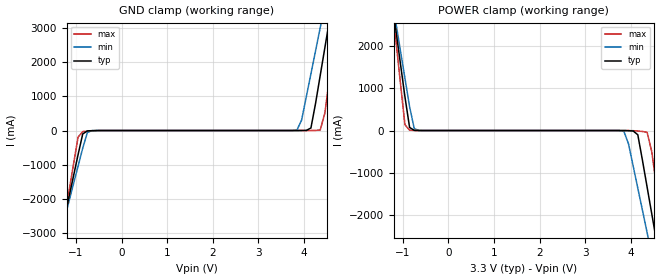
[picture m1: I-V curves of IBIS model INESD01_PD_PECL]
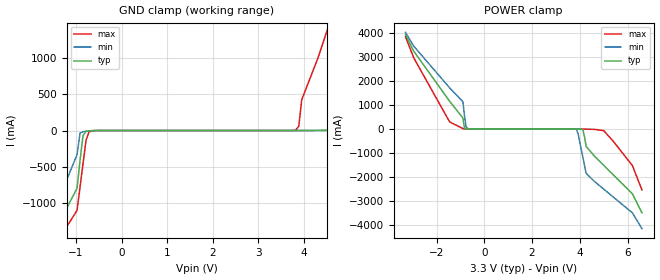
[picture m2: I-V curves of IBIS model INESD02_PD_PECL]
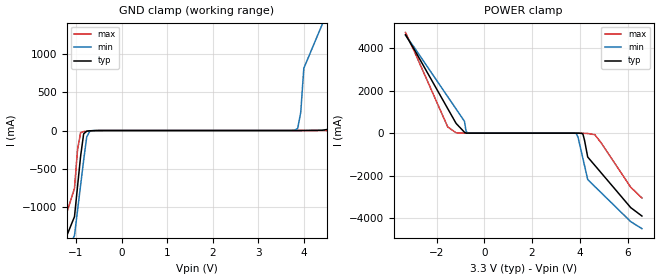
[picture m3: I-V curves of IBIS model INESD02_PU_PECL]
|   This file is an IBIS representation of the   |
|   Integrated Device Technology, Inc.   |
|   ICS8735-31   |
|   1:5 DIFFERENTIAL-TO-3.3V LVPECL ZERO DELAY CLOCK GENERATOR   |
[IBIS Ver]   4.1
[File name]   8735_31_3v3.ibs
[File Rev]   1.1
[Date]   19 Mar 2009 | Last modified
|   Dec 30 2002 | Generated
[Source]   Originated at Integrated Devices Technology, Inc.
[Disclaimer]
IDT hereby grants the user of this IBIS model a non-exclusive,
nontransferable license to use this IBIS model under the following terms.
Before using this IBIS model, the user should read this license.
If the user does not accept these terms,  the IBIS model should be
returned to IDT within 30 days.
   The user is granted this license only to use the IBIS model and
is not granted rights to sell, load, rent, lease or license the IBIS
model in whole or in part, or in modified form to anyone other than
user. User may modify the IBIS model to suit its specific
applications but rights to derivative works and such modifications
shall belong to IDT.
   This IBIS model is provided on an "AS IS" basis and IDT makes
absolutely no warranty with respect to the information contained
herein. IDT DISCLAIMS AND CUSTOMER WAIVES ALL WARRANTIES, EXPRESS
OR IMPLIED, INCLUDING WARRANTIES OF MERCHANTABILITY OR FITNESS FOR
A PARTICULAR PURPOSE. The entire risk as to quality and performance
is with the Customer. ACCORDINGLY, IN NO EVENT SHALL THE COMPANY BE
LIABLE FOR ANY DAMAGES, WHETHER IN CONTRACT OR TORT,INCLUDING ANY
LOST PROFITS OR OTHER INCIDENTAL, CONSEQUENTIAL, EXEMPLARY, OR
PUNITIVE DAMAGES ARISING OUT OF THE USE OR APPLICATION OF THE IBIS
model provided in this package. Further, IDT reserves the right to
make changes without notice to any product herein to improve
reliability, function, or design. IDT does not convey any license
under patent rights or any other intellectual property rights,
including those of third parties.
   IDT is not obligated to provide maintenance or support
for the licensed IBIS model.
[Copyright]   Copyright 2008 by Integrated Device Technology, Inc.
[Component]   ICS8735Y-31
[Manufacturer] Integrated Devices Technology, Inc.
[Package]
|LQFP32
|lead + wire   typ   min   max
R_pkg   220.4m   212.5m   238m
L_pkg   1.841n   1.708n   1.974n
C_pkg   0.316p   0.2907p   0.33p
[Pin] signal_name  model_name   R_pin   L_pin   C_pin
1   SEL0   INESD01_PD_PECL   238m   1.974n   0.330p
2   SEL1   INESD01_PD_PECL   225m   1.841n   0.311p
3   CLK0   INESD02_PD_PECL   218m   1.7745n   0.301p
4   nCLK0   INESD02_PU_PECL   213m   1.708n   0.291p
5   CLK1   INESD02_PD_PECL   213m   1.708n   0.291p
6   nCLK1   INESD02_PU_PECL   218m   1.7745n   0.301p
7   CLK_SEL   INESD01_PD_PECL   225m   1.841n   0.311p
8   MR   INESD01_PD_PECL   238m   1.974n   0.330p
9   VCC   POWER   238m   1.974n   0.330p
10   FB_IN   INESD02_PU_PECL   225m   1.841n   0.311p
11   nFB_IN   INESD02_PD_PECL   218m   1.7745n   0.301p
12   SEL2   INESD01_PD_PECL   213m   1.708n   0.291p
13   VEE   GND   213m   1.708n   0.291p
14   nQ0   ONF01_HSTL01   218m   1.7745n   0.301p
15   Q0   ONF01_HSTL01   225m   1.841n   0.311p
16   VCCO   POWER   238m   1.974n   0.330p
17   VCCO   POWER   238m   1.974n   0.330p
18   nQ1   ONF01_HSTL01   225m   1.841n   0.311p
19   Q1   ONF01_HSTL01   218m   1.7745n   0.301p
20   nQ2   ONF01_HSTL01   213m   1.708n   0.291p
21   Q2   ONF01_HSTL01   213m   1.708n   0.291p
22   nQ3   ONF01_HSTL01   218m   1.7745n   0.301p
23   Q3   ONF01_HSTL01   225m   1.841n   0.311p
24   VCCO   POWER   238m   1.974n   0.330p
25   VCCO   POWER   238m   1.974n   0.330p
26   nQ4   ONF01_HSTL01   225m   1.841n   0.311p
27   Q4   ONF01_HSTL01   218m   1.7745n   0.301p
28   VEE   GND   213m   1.708n   0.291p
29   SEL3   INESD01_PD_PECL   213m   1.708n   0.291p
30   VCCA   POWER   218m   1.7745n   0.301p
31   PLL_SEL   INESD01_PU_PECL   225m   1.841n   0.311p
32   VCC   POWER   238m   1.974n   0.330p
[Diff Pin]  inv_pin  vdiff tdelay_typ tdelay_min  tdelay_max
|Input
3   4   0.15 0  0  0
5   6   0.15 0  0  0
10   11  0.15 0  0  0
|Output
15   14   NA   0  0  0
19   18   NA   0  0  0
21   20   NA   0  0  0
23   22   NA   0  0  0
27   26   NA   0  0  0
| Models and submodels in the file (5): INESD01_PD_PECL (Input), INESD02_PD_PECL (Input), INESD02_PU_PECL (Input), ONF01_HSTL01 (Output_ECL), INESD01_PU_PECL (Input)
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[Model]   INESD01_PD_PECL
Model_type  Input
Polarity   Non-Inverting
Vinl = 0.8V
Vinh = 2.0V
|   typ   min   max
C_comp   2pF   1.5pF   2.5pF
|   typ   min   max
[Voltage range]  3.3V   3.15V   3.45V
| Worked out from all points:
|   GND clamp passes 1 mA (typ) near -0.55 V on its own axis
|   POWER clamp passes 1 mA (typ) near -0.66 V on its own axis
[GND_clamp]
|Voltage   I(typ)   I(min)   I(max)
-2.586V   -10.86A    -9.487A    -13.15A
-1.361V   -3.24A     -3.145A    -3.432A
-1.259V   -2.606A    -2.617A    -2.622A
-952.6mV  -705.3mA   -1.038A    -192.4mA
-850.5mV  -99.9mA    -513.5mA   -31.23mA
-646.4mV  -3.788mA   -3.549mA   -8.297mA
3.844V    129.1uA    13.13mA    71.12uA
4.151V    73.33mA    1.652A     864.7uA
4.355V    1.607A     3.003A     15.44mA
4.559V    3.233A     4.356A     1.553A
4.763V    4.861A     5.711A     3.635A
5.375V    9.757A     9.783A     9.893A
[POWER_clamp]
|Voltage   I(typ)   I(min)   I(max)
-2.177V   10.57A     9.364A     12.62A
-1.157V   2.42A      2.586A     2.194A
-952.6mV  795.8mA    1.237A     137.8mA
-850.5mV  73.33mA    563.2mA    8.145mA
-646.4mV  535.8uA    2.004mA    431.2uA
3.844V    -826.3uA   -18.14mA   -47.07uA
4.151V    -99.9mA    -1.362A    -11.82mA
4.355V    -1.338A    -2.415A    -41.71mA
4.559V    -2.606A    -3.47A     -1.312A
4.661V    -3.24A     -3.998A    -2.123A
4.763V    -3.875A    -4.526A    -2.933A
5.579V    -8.954A    -8.756A    -9.414A
[Model]   INESD02_PD_PECL
Model_type  Input
Polarity   Non-Inverting
Vinl = 0.8V
Vinh = 2.0V
|   typ   min   max
C_comp   2pF   1.5pF   2.5pF
|   typ   min   max
[Voltage range]  3.3V   3.15V   3.45V
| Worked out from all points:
|   GND clamp passes 1 mA (typ) near -0.59 V on its own axis
|   POWER clamp passes 1 mA (typ) near -0.70 V on its own axis
[GND_clamp]
-3.3V     -3.894A    -4.294A    -3.674A
-1.6V     -1.569A    -1.322A    -1.74A
-974.8mV  -794.1mA   -331.5mA   -1.096A
-843.4mV  -68.33mA   -15.34mA   -452.9mA
-646.5mV  -1.912mA   -4.151mA   -2.665mA
3.818V    89.38uA    70.49uA    7.198mA
3.95V     342.2uA    75.94uA    423.8mA
4.6V      7.437mA    165.5uA    1.553A
4.9V      78.32mA    440.9uA    2.118A
5.5V      1.293A     2.769mA    3.249A
6.25V     2.651A     112.4mA    4.38A
6.6V      3.331A     896.1mA    4.946A
[POWER_clamp]
-3.3V     3.923A     4.017A     3.838A
-2.95V    3.23A      3.44A      2.951A
-1.45V    1.149A     1.709A     289.6mA
-896.9mV  456.5mA    1.133A     15.4mA
-762.9mV  4.223mA    91.07mA    1.486mA
-695.9mV  792.2uA    10.73mA    555.6uA
3.861V    -556.7uA   -26.14mA   -39.45uA
4.129V    -41.85mA   -1.19A     -4.904mA
4.263V    -724.2mA   -1.847A    -12.04mA
5V        -1.514A    -2.505A    -71.38mA
6.2V      -2.701A    -3.492A    -1.525A
6.6V      -3.492A    -4.151A    -2.536A
[Model]   INESD02_PU_PECL
Model_type  Input
Polarity   Non-Inverting
Vinl = 0.8V
Vinh = 2.0V
|   typ   min   max
C_comp   2pF   1.5pF   2.5pF
|   typ   min   max
[Voltage range]  3.3V   3.15V   3.45V
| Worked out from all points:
|   GND clamp passes 1 mA (typ) near -0.59 V on its own axis
|   POWER clamp passes 1 mA (typ) near -0.70 V on its own axis
[GND_clamp]
|Voltage   I(typ)   I(min)   I(max)
-3.3V     -3.894A    -3.674A    -4.294A
-1.3V     -1.521A    -1.7A      -1.261A
-1.031V   -1.125A    -1.372A    -755.3mA
-896.9mV  -335.4mA   -714.7mA   -27.07mA
-695.9mV  -3.401mA   -10.69mA   -6.477mA
3.794V    17.99uA    3.319mA    6.081uA
3.928V    181.1uA    239mA      10.12uA
3.995V    711.6uA    813.7mA    20.78uA
4.8V      40.44mA    1.967A     268.6uA
5.6V      1.139A     3.12A      2.243mA
6.3V      2.525A     4.275A     64.01mA
6.6V      3.219A     4.852A     752.7mA
[POWER_clamp]
|Voltage   I(typ)   I(min)   I(max)
-3.3V     4.617A     4.594A     4.726A
-1.53V    1.149A     1.709A     289.6mA
-1.18V    456.4mA    1.132A     15.33mA
-829.9mV  42.02mA    556.1mA    3.39mA
-762.9mV  4.159mA    91mA       1.422mA
-695.9mV  727.9uA    10.66mA    491.6uA
3.861V    -620.9uA   -26.2mA    -103.4uA
4.129V    -41.91mA   -1.19A     -4.968mA
4.33V     -1.119A    -2.176A    -17.93mA
4.63V     -1.515A    -2.505A    -71.45mA
6.13V     -3.492A    -4.151A    -2.536A
6.6V      -3.888A    -4.48A     -3.041A
